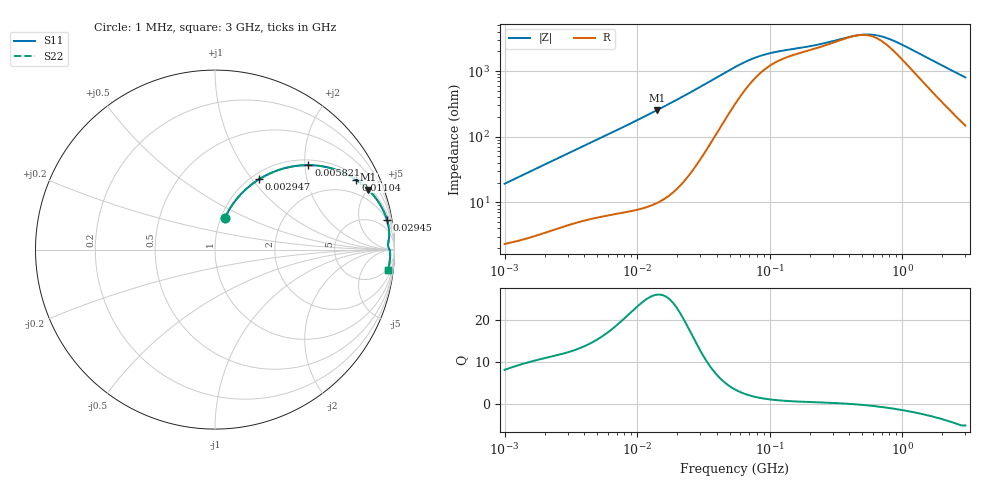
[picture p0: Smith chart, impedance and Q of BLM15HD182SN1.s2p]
! BLM15HD182SN1
# Hz S RI R 50
!Freq.(Hz) S11(Real) S11(Imag) S21(Real) S21(Imag) S12(Real) S12(Imag) S22(Real) S22(Imag)
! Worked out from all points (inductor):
!   401 points, 1 MHz to 3 GHz, reference 50 ohm
!   read as one part in series: L = 3.01 uH near 1.041 MHz
!   highest Q = 26 at 14.04 MHz (marker M1), where L = 2.86 uH
!   self-resonance near 453.8 MHz
!   S11 on the Smith chart (normalised r, x): 1 MHz: 1.05, +0.38; 2.947 MHz: 1.09, +1.08; 5.821 MHz: 1.12, +2.08; 11.04 MHz: 1.16, +3.94; 29.45 MHz: 2, +11; 3 GHz: 4, -16
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1000000  0.0552 0.1755  0.9448 -0.1755  0.9448 -0.1755  0.0552 0.1755
1786863  0.1231 0.2847  0.8769 -0.2847  0.8769 -0.2847  0.1231 0.2847
2947212  0.245 0.3914  0.755 -0.3914  0.755 -0.3914  0.245 0.3914
3823119  0.3376 0.4374  0.6624 -0.4374  0.6624 -0.4374  0.3376 0.4374
5820586  0.5201 0.4707  0.4799 -0.4707  0.4799 -0.4707  0.5201 0.4707
7858845  0.6554 0.4511  0.3446 -0.4511  0.3446 -0.4511  0.6554 0.4511
1.104425e7  0.786 0.3901  0.214 -0.3901  0.214 -0.3901  0.786 0.3901
1.404268e7  0.855 0.3335  0.145 -0.3335  0.145 -0.3335  0.855 0.3335
1.461624e7  0.8645 0.3236  0.1355 -0.3236  0.1355 -0.3236  0.8645 0.3236
2.013356e7  0.9224 0.2464  0.0776 -0.2464  0.0776 -0.2464  0.9224 0.2464
2.944989e7  0.9577 0.167  0.0423 -0.167  0.0423 -0.167  0.9577 0.167
5.477226e7  0.9705 0.0791  0.0295 -0.0791  0.0295 -0.0791  0.9705 0.0791
7.248696e7  0.9684 0.0557  0.0316 -0.0557  0.0316 -0.0557  0.9684 0.0557
9.402997e7  0.9658 0.0409  0.0342 -0.0409  0.0342 -0.0409  0.9658 0.0409
2.094008e8  0.9647 0.0181  0.0353 -0.0181  0.0353 -0.0181  0.9647 0.0181
4.135554e8  0.9713 0.00267  0.0287 -0.00267  0.0287 -0.00267  0.9713 0.00267
5.051982e8  0.9731 -0.0033  0.0269 0.0033  0.0269 0.0033  0.9731 -0.0033
6.296259e8  0.9747 -0.0108  0.0253 0.0108  0.0253 0.0108  0.9747 -0.0108
8.005644e8  0.9757 -0.0202  0.0243 0.0202  0.0243 0.0202  0.9757 -0.0202
1.017911e9  0.976 -0.0312  0.024 0.0312  0.024 0.0312  0.976 -0.0312
1.645649e9  0.9742 -0.0598  0.0258 0.0598  0.0258 0.0598  0.9742 -0.0598
3e9  0.9638 -0.1156  0.0362 0.1156  0.0362 0.1156  0.9638 -0.1156
